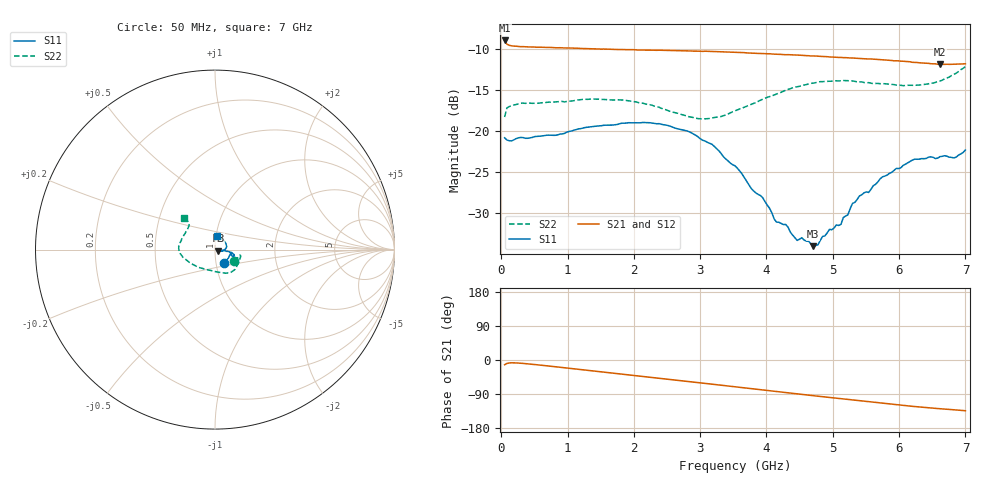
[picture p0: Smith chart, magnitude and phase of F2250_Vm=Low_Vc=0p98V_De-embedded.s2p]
! Integrated Device Technology
! Corporate Headquarters
! 6024 Silver Creek Valley Road
! San Jose, CA 95138  USA
! Phone:  1-408-284-8200
! Toll Free:  1-800-223-1366
! Webpage:  http://www.idt.com/
! Timing and RF Division
! 515 Groton Road, Suite 102
! Westford, MA 01886-6024
! Device:  F2250
! Description: Voltage Variable RF Attenuator
! Frequency:  50.0 -  6000.00 MHz
! Package:  3x3 mm Thin QFN Plastic Package: 16 pin
! Ports:  2 RF, 3 DC
!  Pin  1  = GND
!  Pin  2  = NC
!  Pin  3  = RF1  = Port 1
!  Pin  4  = NC
!  Pin  5  = GND
!  Pin  6  = GND
!  Pin  7  = GND
!  Pin  8  = GND
!  Pin  9  = NC
!  Pin 10  = RF2  = Port 2
!  Pin 11  = NC
!  Pin 12  = GND
!  Pin 13  = GND
!  Pin 14  = VCNTRL
!  Pin 15  = VDD
!  Pin 16  = VMODE
! Vcntrl:  0.980 Volts
! Vmode:  +0.000 Volts
! Vdd:  +3.30  Volts
! Current:  1.185 mA
! Data:  The device was measured on a the F2250 evaluation board which has
!  individual transmission lines to the RF pins.  Data was collected
!  using a calibrated network analyzer.  The evaluation board was
!  de-embedded using a TRL calibration technique.
!  The reference plane is the edge of the package pin.
! Misc:  SN 10
!  Action Tracker AT0258
! Date Measured:  2014-11-26
! Date:  2015-10-15  MJV
! Note:
!  Integrated Device Technology supplies this data as a sample of measured
!  data at the package pin for this product.  Your particular data for this
!  product may vary.
!  Data was taken at 25 degrees C.
!  Integrated Device Technology reserves the right to change this data at anytime.
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# GHz S dB R 50
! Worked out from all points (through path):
!   201 points, 50 MHz to 7 GHz, reference 50 ohm
!   highest |S21| = -8.97 dB at 50 MHz (marker M1); lowest = -11.9 dB at 6.618 GHz (marker M2)
!   group delay of S21, straight-line fit = 53.4 ps
!   lowest |S11| = -34.0 dB at 4.707 GHz (marker M3), VSWR 1.04, Z = 52 - j0.545 ohm
!   |S11| at or under -10 dB: start of sweep to end of sweep
!   |S22| runs from -18.5 to -12.1 dB; largest |S21 - S12| = 0.0014
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0.05  -20.81 -56.6  -8.97 -12.5  -8.97 -12.5  -18.28 -31.1
0.08475  -21.08 -31.5  -9.43 -9.0  -9.42 -9.0  -17.18 -17.0
0.29325  -20.76 -12.6  -9.73 -8.5  -9.71 -8.5  -16.61 -14.4
1.2315  -19.63 -20.5  -9.96 -25.8  -9.97 -25.8  -16.13 -41.7
2.37825  -19.09 -15.9  -10.16 -47.8  -10.15 -47.9  -17.09 -69.3
3.0385  -21.11 -10.0  -10.30 -61.0  -10.27 -61.0  -18.53 -101.3
3.525  -24.22 -8.2  -10.41 -70.8  -10.42 -70.8  -17.53 -131.2
3.76825  -26.95 -6.9  -10.51 -75.6  -10.50 -75.6  -16.74 -143.4
3.942  -28.09 -7.9  -10.56 -79.0  -10.57 -79.0  -16.13 -151.1
4.1505  -31.06 -9.7  -10.65 -83.2  -10.64 -83.2  -15.49 -159.2
4.2895  -31.34 -12.3  -10.71 -85.9  -10.69 -85.9  -15.02 -163.6
4.46325  -33.28 -15.1  -10.74 -89.4  -10.75 -89.4  -14.60 -168.3
4.53275  -32.96 -13.8  -10.79 -90.8  -10.80 -90.8  -14.45 -170.3
4.7065  -33.99 -15.2  -10.85 -94.2  -10.85 -94.2  -14.16 -174.1
4.94975  -31.94 -16.6  -10.98 -98.9  -10.97 -98.9  -13.93 -179.4
5.1235  -31.33 -16.4  -11.04 -102.3  -11.03 -102.3  -13.88 176.6
5.4015  -27.88 -9.2  -11.16 -107.5  -11.16 -107.5  -14.01 170.0
5.85325  -25.13 0.2  -11.39 -116.0  -11.39 -116.1  -14.31 158.5
6.2355  -23.40 15.6  -11.64 -122.8  -11.64 -122.9  -14.43 145.9
6.61775  -23.10 39.5  -11.89 -128.5  -11.87 -128.6  -13.90 135.4
6.82625  -23.26 59.5  -11.85 -131.4  -11.85 -131.4  -13.10 134.1
7  -22.29 82.9  -11.81 -133.9  -11.82 -134.0  -12.15 134.1
